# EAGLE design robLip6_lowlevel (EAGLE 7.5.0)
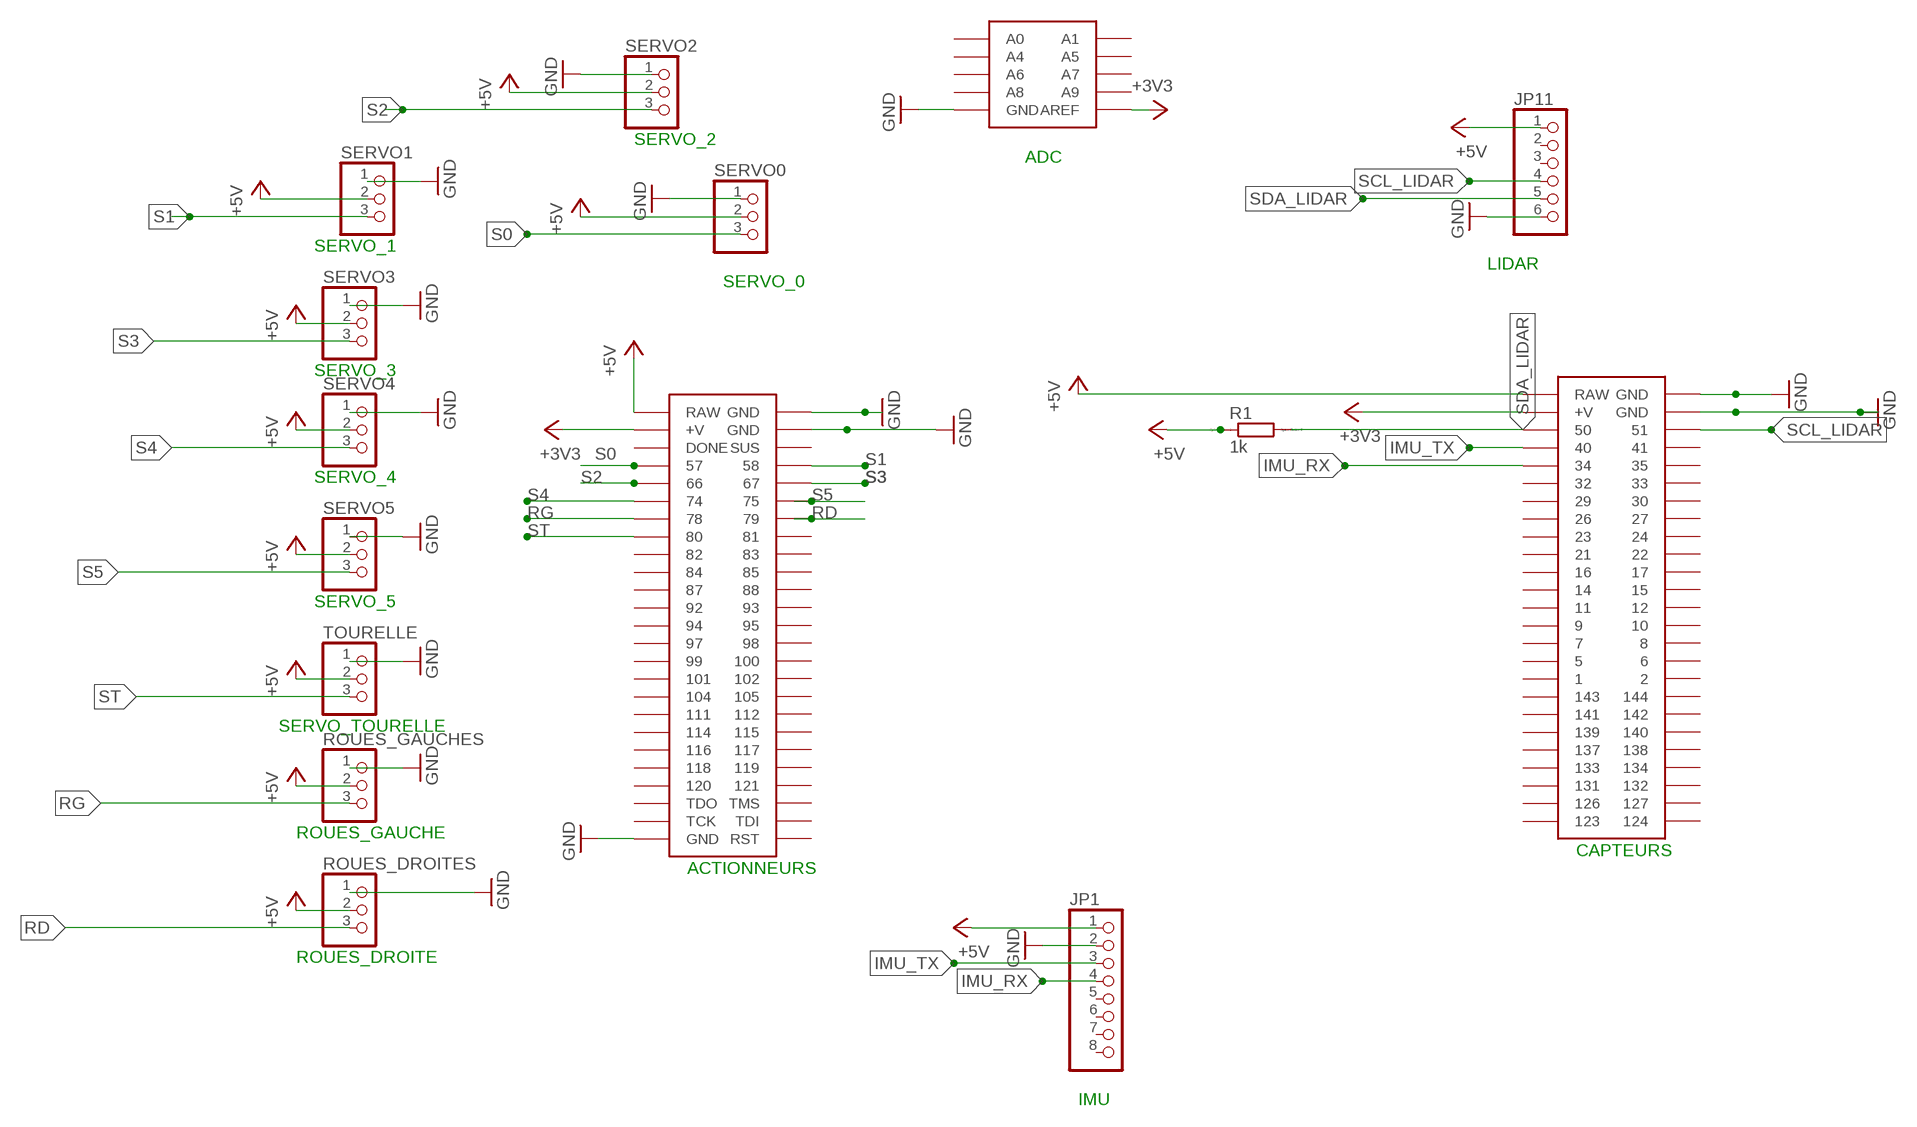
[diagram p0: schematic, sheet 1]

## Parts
JP1  PINHD-1X8  [1X08]
JP11  PINHD-1X6  [1X06]
R1  1k  R0207/10  [0207/10]
ROUES_DROITES  PINHD-1X3/90  [1X03/90]
ROUES_GAUCHES  PINHD-1X3/90  [1X03/90]
SERVO0  PINHD-1X3/90  [1X03/90]
SERVO1  PINHD-1X3/90  [1X03/90]
SERVO2  PINHD-1X3/90  [1X03/90]
SERVO3  PINHD-1X3/90  [1X03/90]
SERVO4  PINHD-1X3/90  [1X03/90]
SERVO5  PINHD-1X3/90  [1X03/90]
TOURELLE  PINHD-1X3/90  [1X03/90]
U$1  MOJOV3  [MOJO_V3]

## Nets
+3V3: U$1.AREF U$1.V@1(+V) U$1.V@2(+V)
+5V: JP1.1 JP11.1 R1.1 ROUES_DROITES.2 ROUES_GAUCHES.2 SERVO0.2 SERVO1.2 SERVO2.2 SERVO3.2 SERVO4.2 SERVO5.2 TOURELLE.2 U$1.RAW@1(RAW)
GND: JP1.2 JP11.6 ROUES_DROITES.1 ROUES_GAUCHES.1 SERVO0.1 SERVO1.1 SERVO2.1 SERVO3.1 SERVO4.1 SERVO5.1 TOURELLE.1 U$1.GND@2(GND) U$1.GND@3(GND) U$1.GND@4(GND) U$1.GND@5(GND) U$1.GND@6(GND)
GND@1: U$1.GND@1(GND) ; supply symbol labelled GND
IMU_RX: JP1.4 U$1.34
IMU_TX: JP1.3 U$1.40
RAW: U$1.RAW@2(RAW) ; supply symbol labelled +5V
RD: ROUES_DROITES.3 U$1.79
RG: ROUES_GAUCHES.3 U$1.78
S0: SERVO0.3 U$1.57
S1: SERVO1.3 U$1.58
S2: SERVO2.3 U$1.66
S3: SERVO3.3 U$1.67
S4: SERVO4.3 U$1.74
S5: SERVO5.3 U$1.75
SCL_LIDAR: JP11.4 U$1.51
SDA_LIDAR: JP11.5 R1.2 U$1.50
ST: TOURELLE.3 U$1.80
Unconnected: JP1.5 JP1.6 JP1.7 JP1.8 JP11.2 JP11.3 U$1.1 U$1.2 U$1.5 U$1.6 U$1.7 U$1.8 U$1.9 U$1.10 U$1.11 U$1.12 U$1.14 U$1.15 U$1.16 U$1.17 U$1.21 U$1.22 U$1.23 U$1.24 U$1.26 U$1.27 U$1.29 U$1.30 U$1.32 U$1.33 U$1.35 U$1.41 U$1.81 U$1.82 U$1.83 U$1.84 U$1.85 U$1.87 U$1.88 U$1.92 U$1.93 U$1.94 U$1.95 U$1.97 U$1.98 U$1.99 U$1.100 U$1.101 U$1.102 U$1.104 U$1.105 U$1.111 U$1.112 U$1.114 U$1.115 U$1.116 U$1.117 U$1.118 U$1.119 U$1.120 U$1.121 U$1.123 U$1.124 U$1.126 U$1.127 U$1.131 U$1.132 U$1.133 U$1.134 U$1.137 U$1.138 U$1.139 U$1.140 U$1.141 U$1.142 U$1.143 U$1.144 U$1.A0 U$1.A1 U$1.A4 U$1.A5 U$1.A6 U$1.A7 U$1.A8 U$1.A9 U$1.DONE U$1.RST U$1.SUS U$1.TCK U$1.TDI U$1.TDO U$1.TMS

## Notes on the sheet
- SERVO_2
- ADC
- SERVO_1
- LIDAR
- SERVO_0
- SERVO_3
- SERVO_4
- SERVO_5
- SERVO_TOURELLE
- ROUES_GAUCHE
- CAPTEURS
- ACTIONNEURS
- ROUES_DROITE
- IMU

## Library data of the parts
JP1 = pinhead:PINHD-1X8: PIN HEADER
JP11 = pinhead:PINHD-1X6: PIN HEADER
R1 = eagle-ltspice:R: RESISTOR, European symbol; SPICEMODEL: NONE; SPICEPREFIX: R
ROUES_DROITES ROUES_GAUCHES SERVO0 SERVO1-SERVO5 TOURELLE = pinhead:PINHD-1X3: PIN HEADER
U$1 = EmbeddedMicro-Mojo:MOJO

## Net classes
0 default: width 0.305 mm, drill 0.508 mm, clearance 0.254 mm

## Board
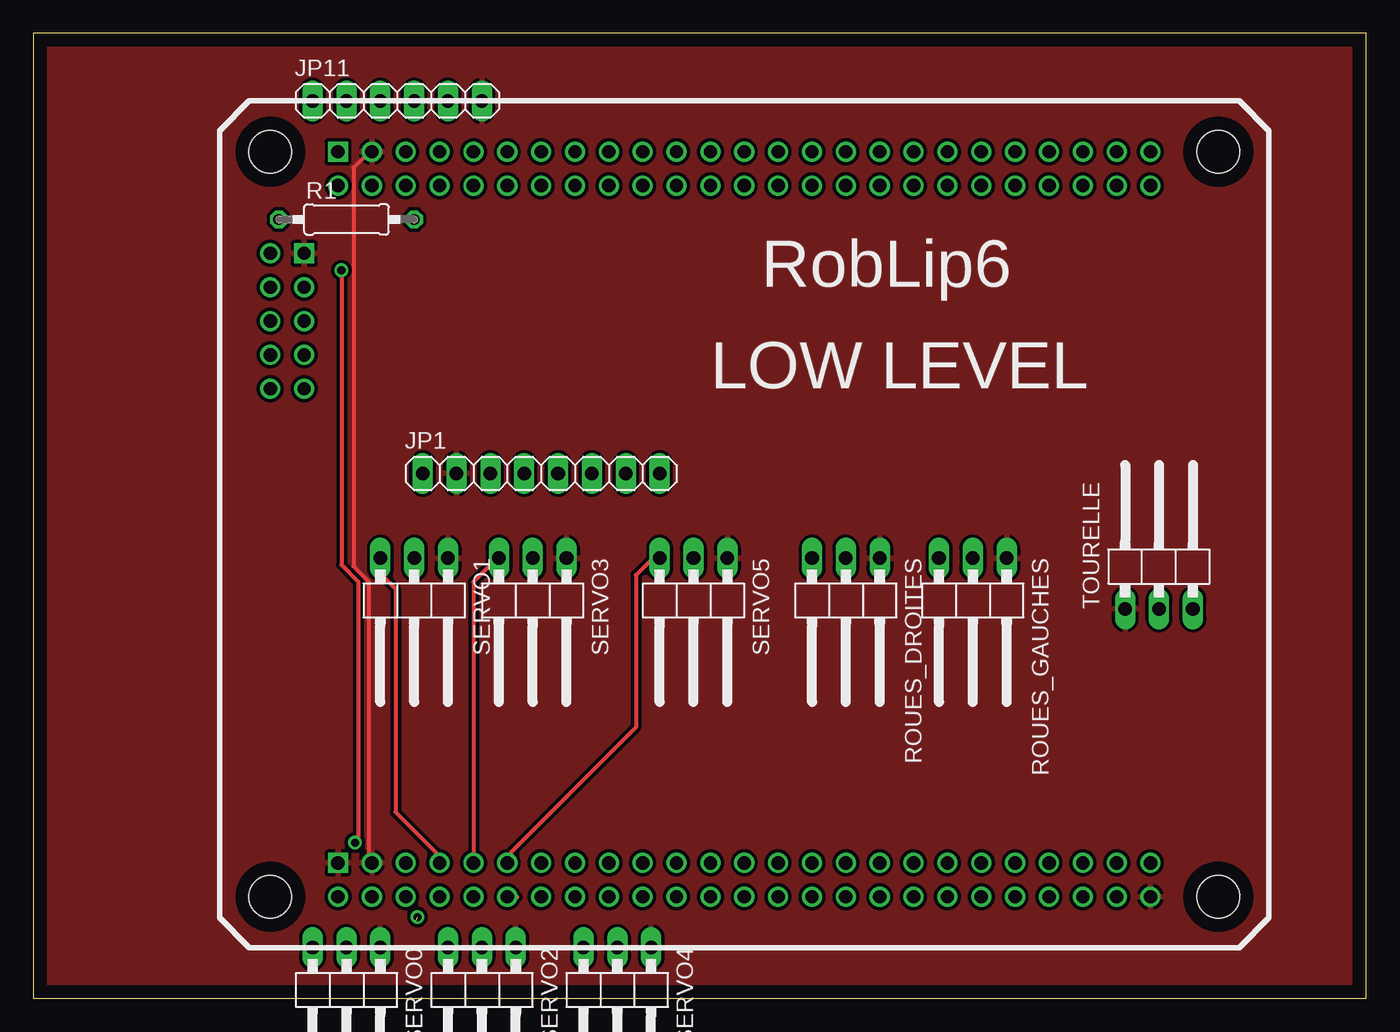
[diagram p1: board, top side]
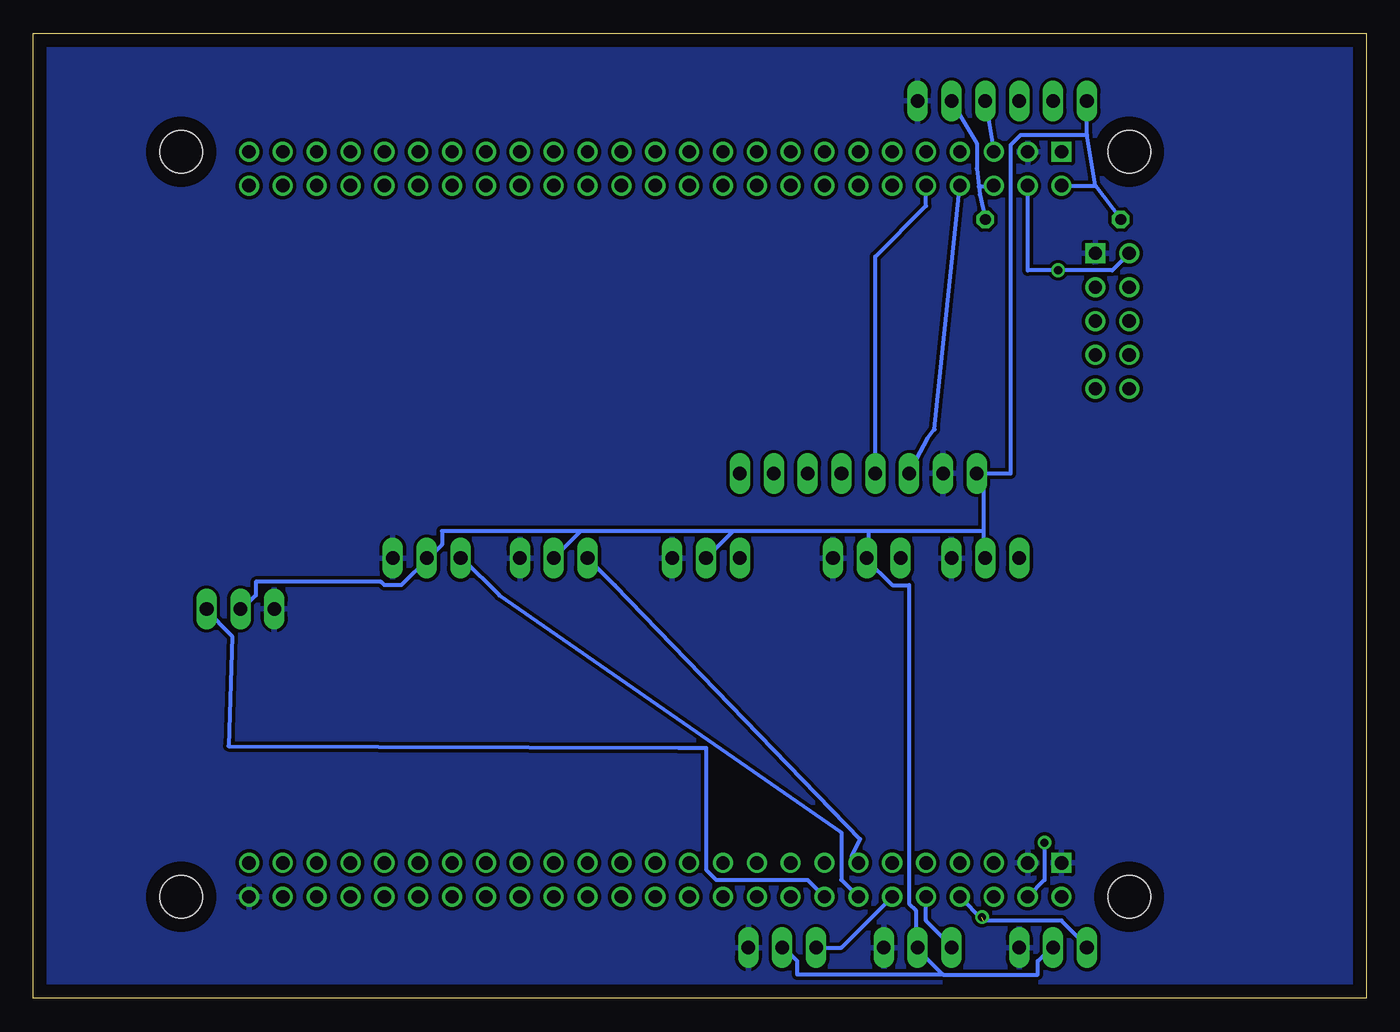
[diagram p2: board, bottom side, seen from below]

Size 100 x 72.38 mm. Coordinates in mm from the lower left corner, seen from the top.
Outline: 0,0 100,0 100,72.38 0,72.38 0,0
Copper layers (1*16): Top 0.035mm / dielectric 1.5mm / Bottom 0.035mm
Design rules "default *": minimum track width 10mil, minimum drill 24mil, track to track 8mil, track to pad 8mil, pad to pad 8mil, via to via 8mil, smd to smd 8mil, copper to edge 40mil, drill to drill 8mil, minimum pad ring 10mil, minimum via ring 8mil, stop-mask expansion 4mil, vias tented up to drill 0mil, thermal gap 10mil

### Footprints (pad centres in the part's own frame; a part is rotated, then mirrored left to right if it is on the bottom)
1X08 = drill 1.016 long: 1 -8.89,0; 2 -6.35,0; 3 -3.81,0; 4 -1.27,0; 5 1.27,0; 6 3.81,0; 7 6.35,0; 8 8.89,0
1X06 = drill 1.016 long: 1 -6.35,0; 2 -3.81,0; 3 -1.27,0; 4 1.27,0; 5 3.81,0; 6 6.35,0
0207/10 = drill 0.813 octagon: 1 -5.08,0; 2 5.08,0
1X03/90 = drill 1.016 long: 1 -2.54,-3.81; 2 0,-3.81; 3 2.54,-3.81
MOJO_V3 = drill 1: 1 49.53,57.15; 2 49.53,59.69; 5 46.99,57.15; 6 46.99,59.69; 7 44.45,57.15; 8 44.45,59.69; 9 41.91,57.15; 10 41.91,59.69; 11 39.37,57.15; 12 39.37,59.69; 14 36.83,57.15; 15 36.83,59.69; 16 34.29,57.15; 17 34.29,59.69; 21 31.75,57.15; 22 31.75,59.69; 23 29.21,57.15; 24 29.21,59.69; 26 26.67,57.15; 27 26.67,59.69; 29 24.13,57.15; 30 24.13,59.69; 32 21.59,57.15; 33 21.59,59.69; 34 19.05,57.15; 35 19.05,59.69; 40 16.51,57.15; 41 16.51,59.69; 50 13.97,57.15; 51 13.97,59.69; 57 16.51,3.81; 58 16.51,6.35; 66 19.05,3.81; 67 19.05,6.35; 74 21.59,3.81; 75 21.59,6.35; 78 24.13,3.81; 79 24.13,6.35; 80 26.67,3.81; 81 26.67,6.35; 82 29.21,3.81; 83 29.21,6.35; 84 31.75,3.81; 85 31.75,6.35; 87 34.29,3.81; 88 34.29,6.35; 92 36.83,3.81; 93 36.83,6.35; 94 39.37,3.81; 95 39.37,6.35; 97 41.91,3.81; 98 41.91,6.35; 99 44.45,3.81; 100 44.45,6.35; 101 46.99,3.81; 102 46.99,6.35; 104 49.53,3.81; 105 49.53,6.35; 111 52.07,3.81; 112 52.07,6.35; 114 54.61,3.81; 115 54.61,6.35; 116 57.15,3.81; 117 57.15,6.35; 118 59.69,3.81; 119 59.69,6.35; 120 62.23,3.81; 121 62.23,6.35; 123 69.85,57.15; 124 69.85,59.69; 126 67.31,57.15; 127 67.31,59.69; 131 64.77,57.15; 132 64.77,59.69; 133 62.23,57.15; 134 62.23,59.69; 137 59.69,57.15; 138 59.69,59.69; 139 57.15,57.15; 140 57.15,59.69; 141 54.61,57.15; 142 54.61,59.69; 143 52.07,57.15; 144 52.07,59.69; A0 6.35,41.91; A1 3.81,41.91; A4 6.35,44.45; A5 3.81,44.45; A6 6.35,46.99; A7 3.81,46.99; A8 6.35,49.53; A9 3.81,49.53; AREF 3.81,52.07; DONE 13.97,3.81; GND@2 11.43,59.69; GND@4 11.43,6.35; GND@6 69.85,3.81; RAW@1 8.89,57.15; RAW@2 8.89,3.81; RST 69.85,6.35; SUS 13.97,6.35; TCK 67.31,3.81; TDI 67.31,6.35; TDO 64.77,3.81; TMS 64.77,6.35; V@1 11.43,57.15; V@2 11.43,3.81 | drill 1 square: GND@1 8.89,59.69; GND@3 8.89,6.35; GND@5 6.35,52.07 | hole 3.2: 3.81,3.81; 3.81,59.69; 74.93,59.69; 74.93,3.81

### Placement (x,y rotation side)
JP1  38.1,39.37 0 top
JP11  27.3,67.31 0 top
R1  23.5,58.42 0 top
ROUES_DROITES  60.96,29.21 180 top
ROUES_GAUCHES  70.48,29.21 180 top
SERVO0  23.5,0 180 top
SERVO1  28.57,29.21 180 top
SERVO2  33.66,0 180 top
SERVO3  37.47,29.21 180 top
SERVO4  43.81,0 180 top
SERVO5  49.53,29.21 180 top
TOURELLE  84.45,33.02 0 top
U$1  13.97,3.81 0 top

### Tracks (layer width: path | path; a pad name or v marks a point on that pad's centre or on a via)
+3V3  (via drill 0.61)
  Top 0.305: v24.13,11.68 24.38,11.94 24.38,31.24 23.11,32.51 v23.11,54.61
  Bottom 0.305: U$1.AREF 19.05,54.61 v23.11,54.61 25.4,54.61 U$1.V@1 | U$1.V@2 24.13,8.89 v24.13,11.68
+5V
  Bottom 0.305: U$1.RAW@1 20.32,60.96 | 20.32,60.96 R1.1 | 20.32,60.96 20.95,64.77 | 20.95,64.77 JP11.1 | 28.7,39.37 28.7,35.05 | 28.7,35.05 28.7,33.02 SERVO1.2 28.45,33.02 | 37.34,35.05 37.34,33.02 SERVO3.2 37.59,33.02 35.56,30.99 34.29,30.99 34.29,7.11 33.78,6.6 33.78,3.81 | 28.7,35.05 37.34,35.05 | 47.5,35.05 SERVO5.2 | 37.34,35.05 47.5,35.05 | 58.93,35.05 ROUES_DROITES.2 | 47.5,35.05 58.93,35.05 | 20.95,64.77 25.91,64.77 26.67,64.01 26.67,39.37 28.7,39.37 | 28.7,39.37 JP1.1 | 31.75,1.78 24.64,1.78 24.64,2.79 23.62,3.81 SERVO0.2 | 33.78,3.81 31.75,1.78 | 31.75,1.78 42.67,1.78 42.67,2.79 43.69,3.81 SERVO4.2 | 70.36,33.02 72.39,30.99 73.66,30.99 73.91,31.24 83.31,31.24 83.31,30.23 84.33,29.21 TOURELLE.2 | 70.36,33.02 69.34,34.04 69.34,35.05 58.93,35.05 | 70.36,33.02 ROUES_GAUCHES.2 | 33.78,3.81 SERVO2.2
GND
  Top 0.305: 25.15,10.34 25.15,31.29 24.03,32.41 24.03,62.31 25.15,63.42 U$1.GND@2
  pour Top: -1.27,73.66 -1.27,-1.27 101.6,-1.27 101.6,73.66
  pour Bottom: -1.27,73.66 -1.27,-1.27 101.6,-1.27 101.6,73.66
IMU_RX
  Bottom 0.305: U$1.34 33.02,59.44 36.83,55.63 JP1.4
IMU_TX
  Bottom 0.305: U$1.40 32.38,42.67 32.89,42.04 JP1.3
RD
  Bottom 0.305: U$1.79 38.61,10.67 37.97,11.94 56.39,30.99 ROUES_DROITES.3
RG
  Bottom 0.305: U$1.78 39.37,8.89 39.37,12.45 65.02,30.23 67.82,33.02 ROUES_GAUCHES.3
S0  (via drill 0.61)  (1 unrouted)
  Bottom 0.305: U$1.57 28.7,5.84 22.86,5.84 20.83,3.81 SERVO0.3
  other vias: 28.83,6.1
S1
  Top 0.305: U$1.58 30.23,10.41 30.23,10.92 27.18,13.97 27.18,30.73 26.16,31.75 26.16,33.02 SERVO1.3
  Bottom 0.305: 25.91,33.02 SERVO1.3
S2
  Bottom 0.305: U$1.66 33.02,5.84 30.99,3.81 SERVO2.3
S3
  Top 0.305: U$1.67 33.02,31.24 34.8,33.02 SERVO3.3
S4
  Top 0.305: 36.32,7.62 U$1.74
  Bottom 0.305: U$1.74 39.37,3.81 SERVO4.3
S5
  Top 0.305: U$1.75 35.81,10.41 35.81,10.92 45.21,20.32 45.21,31.75 46.48,33.02 SERVO5.3
SCL_LIDAR
  Bottom 0.305: JP11.4 U$1.51
SDA_LIDAR
  Bottom 0.305: 28.99,60.28 29.21,62.23 29.21,64.14 JP11.5 | 28.99,60.28 R1.2 | U$1.50 27.94,60.91 29.06,60.91 28.99,60.28
ST
  Bottom 0.305: U$1.80 41.91,8.89 48.77,8.89 49.53,9.65 49.53,18.8 51.56,18.8 85.34,18.92 85.09,27.18 87.12,29.21 TOURELLE.3

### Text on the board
tNames: RobLip6 | LOW LEVEL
